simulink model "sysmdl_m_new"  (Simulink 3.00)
settings: Solver=ode23s  SolverMode=SingleTasking  StartTime=0.0  StopTime=50.0  RelTol=1e-3  AbsTol=1e-6
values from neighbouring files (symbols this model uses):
  c = fminsearch('pdn_prf',k,options)    [optimise.m]    (also in optimise_new.m = fminsearch('pdn_prf_new',k,options))

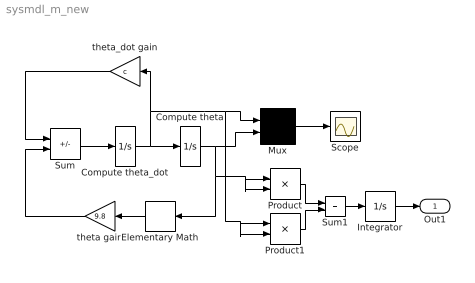
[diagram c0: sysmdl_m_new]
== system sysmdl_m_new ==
  Compute theta : Integrator  ExternalReset=none  InitialConditionSource=internal  InitialCondition=pi/3  LimitOutput=off  UpperSaturationLimit=inf  LowerSaturationLimit=-inf  ShowSaturationPort=off  ShowStatePort=off  AbsoluteTolerance=auto
  Compute theta_dot : Integrator  ExternalReset=none  InitialConditionSource=internal  InitialCondition=0  LimitOutput=off  UpperSaturationLimit=inf  LowerSaturationLimit=-inf  ShowSaturationPort=off  ShowStatePort=off  AbsoluteTolerance=auto
  Elementary Math : ElementaryMath  Orientation=left  Operator=sin
  Integrator : Integrator  ExternalReset=none  InitialConditionSource=internal  InitialCondition=0  LimitOutput=off  UpperSaturationLimit=inf  LowerSaturationLimit=-inf  ShowSaturationPort=off  ShowStatePort=off  AbsoluteTolerance=auto
  Mux : Mux  Inputs=2
  Product : Product  Inputs=2  SaturateOnIntegerOverflow=on
  Product1 : Product  Inputs=2  SaturateOnIntegerOverflow=on
  Scope : Scope
  Sum : Sum  Inputs=--  SaturateOnIntegerOverflow=on
  Sum1 : Sum  Inputs=|++  SaturateOnIntegerOverflow=on
  theta gain : Gain  Orientation=left  Gain=9.8  SaturateOnIntegerOverflow=on
  theta_dot gain : Gain  Orientation=left  Gain=c  SaturateOnIntegerOverflow=on
  Out1 : Outport  Port=1
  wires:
  Compute theta_dot/1 -> Compute theta/1, theta_dot gain/1, Mux/1, Product1/1, Product1/2
  Sum/1 -> Compute theta_dot/1
  theta_dot gain/1 -> Sum/1
  Mux/1 -> Scope/1
  Compute theta/1 -> Mux/2, Elementary Math/1, Product/1, Product/2
  Elementary Math/1 -> theta gain/1
  theta gain/1 -> Sum/2
  Product/1 -> Sum1/1
  Product1/1 -> Sum1/2
  Sum1/1 -> Integrator/1
  Integrator/1 -> Out1/1
